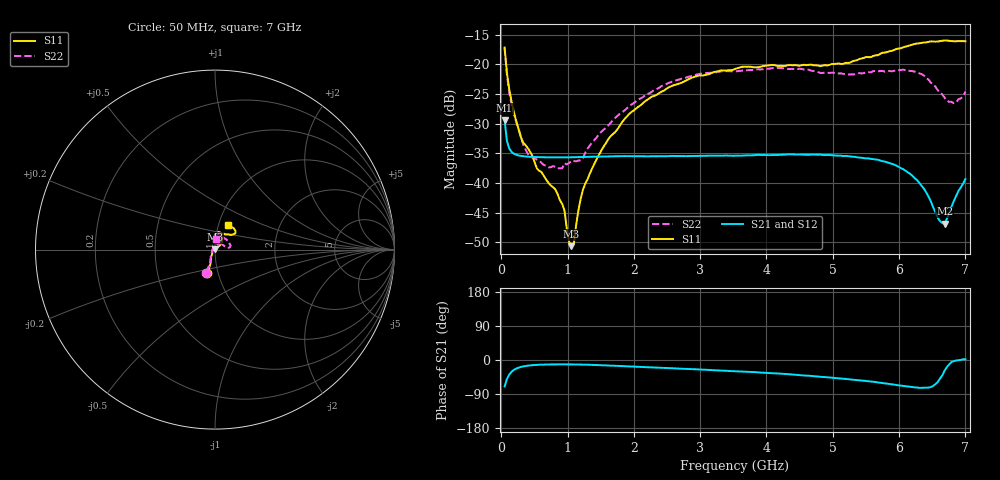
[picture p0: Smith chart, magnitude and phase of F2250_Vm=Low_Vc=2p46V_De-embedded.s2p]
! Integrated Device Technology
! Corporate Headquarters
! 6024 Silver Creek Valley Road
! San Jose, CA 95138  USA
! Phone:  1-408-284-8200
! Toll Free:  1-800-223-1366
! Webpage:  http://www.idt.com/
! Timing and RF Division
! 515 Groton Road, Suite 102
! Westford, MA 01886-6024
! Device:  F2250
! Description: Voltage Variable RF Attenuator
! Frequency:  50.0 -  6000.00 MHz
! Package:  3x3 mm Thin QFN Plastic Package: 16 pin
! Ports:  2 RF, 3 DC
!  Pin  1  = GND
!  Pin  2  = NC
!  Pin  3  = RF1  = Port 1
!  Pin  4  = NC
!  Pin  5  = GND
!  Pin  6  = GND
!  Pin  7  = GND
!  Pin  8  = GND
!  Pin  9  = NC
!  Pin 10  = RF2  = Port 2
!  Pin 11  = NC
!  Pin 12  = GND
!  Pin 13  = GND
!  Pin 14  = VCNTRL
!  Pin 15  = VDD
!  Pin 16  = VMODE
! Vcntrl:  2.460 Volts
! Vmode:  +0.000 Volts
! Vdd:  +3.30  Volts
! Current:  1.175 mA
! Data:  The device was measured on a the F2250 evaluation board which has
!  individual transmission lines to the RF pins.  Data was collected
!  using a calibrated network analyzer.  The evaluation board was
!  de-embedded using a TRL calibration technique.
!  The reference plane is the edge of the package pin.
! Misc:  SN 10
!  Action Tracker AT0258
! Date Measured:  2014-11-26
! Date:  2015-10-15  MJV
! Note:
!  Integrated Device Technology supplies this data as a sample of measured
!  data at the package pin for this product.  Your particular data for this
!  product may vary.
!  Data was taken at 25 degrees C.
!  Integrated Device Technology reserves the right to change this data at anytime.
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# GHz S dB R 50
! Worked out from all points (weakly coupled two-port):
!   201 points, 50 MHz to 7 GHz, reference 50 ohm
!   highest |S21| = -29.41 dB at 50 MHz (marker M1); lowest = -46.9 dB at 6.687 GHz (marker M2)
!   lowest |S11| = -50.6 dB at 1.058 GHz (marker M3), VSWR 1.01, Z = 49.8 + j0.244 ohm
!   |S11| at or under -10 dB: start of sweep to end of sweep
!   |S22| runs from -37.5 to -17.3 dB; largest |S21 - S12| = 5.6e-05
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0.05  -17.18 -108.6  -29.41 -69.8  -29.41 -69.8  -17.28 -111.0
0.08475  -21.44 -107.4  -32.92 -50.4  -32.92 -50.3  -21.75 -110.2
0.15425  -26.23 -116.6  -34.75 -31.2  -34.75 -31.1  -26.81 -122.4
0.29325  -32.21 -127.8  -35.43 -18.5  -35.43 -18.5  -32.09 -137.5
0.3975  -34.08 -141.8  -35.56 -15.0  -35.56 -15.0  -35.04 -160.5
0.5365  -37.56 -155.7  -35.64 -12.8  -35.63 -12.8  -36.05 178.1
0.91875  -43.52 157.9  -35.69 -11.5  -35.68 -11.5  -37.52 133.5
0.9535  -44.66 169.8  -35.68 -11.5  -35.68 -11.5  -36.66 131.1
1.023  -49.91 143.5  -35.67 -11.6  -35.68 -11.6  -36.62 116.0
1.05775  -50.64 123.5  -35.67 -11.6  -35.67 -11.6  -36.27 110.8
1.0925  -50.36 89.4  -35.66 -11.7  -35.66 -11.7  -36.30 106.2
1.162  -44.68 56.8  -35.64 -11.9  -35.64 -11.9  -36.21 95.5
1.2315  -41.12 44.2  -35.61 -12.1  -35.61 -12.1  -35.79 85.9
1.6485  -32.11 42.0  -35.52 -14.6  -35.52 -14.7  -29.88 64.6
2.37825  -24.88 47.4  -35.48 -20.3  -35.48 -20.3  -23.99 56.9
3.525  -20.80 72.4  -35.41 -29.5  -35.40 -29.5  -21.19 74.8
4.7065  -20.17 72.3  -35.20 -42.5  -35.20 -42.5  -21.14 72.3
5.85325  -17.81 40.5  -36.64 -63.3  -36.64 -63.3  -21.13 23.0
6.27025  -16.51 40.0  -39.50 -72.6  -39.51 -72.6  -21.35 9.6
6.68725  -15.99 48.8  -46.86 -27.7  -46.83 -27.3  -25.64 28.5
6.861  -16.13 55.1  -42.18 -1.3  -42.14 -1.2  -26.46 58.0
7  -16.12 63.2  -39.34 1.9  -39.30 1.8  -24.63 83.1
